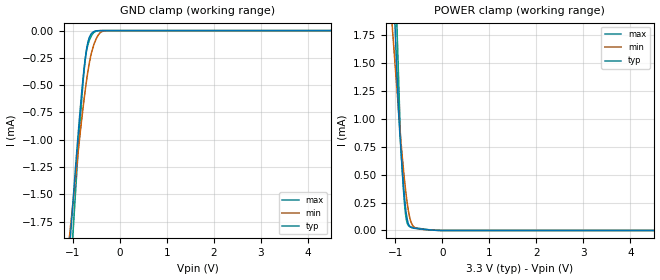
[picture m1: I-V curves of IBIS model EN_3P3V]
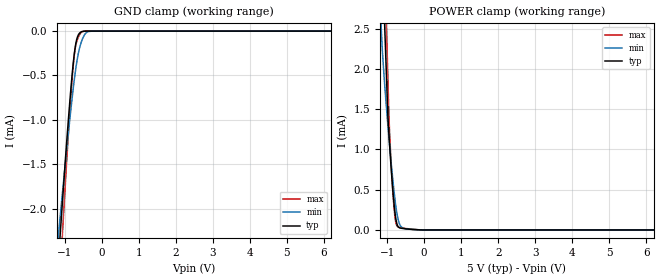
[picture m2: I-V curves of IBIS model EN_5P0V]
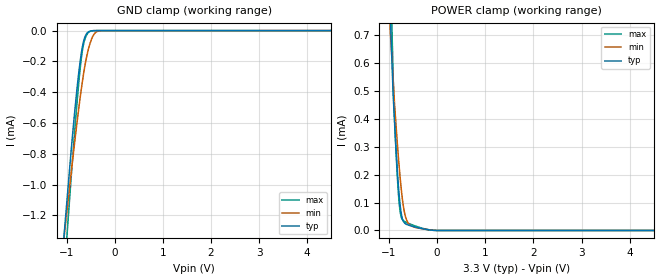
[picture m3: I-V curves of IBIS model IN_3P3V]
| Texas Instruments Incorporated
| Low-Power Quad-channel Digital Isolator
| Marketing part#   Voltage Range   Package-type   #pins/pkg drawing
| ISO7342CDW   3.0V - 5.5V   SOIC   16-pin DW
| ISO7342CDWR   3.0V - 5.5V   SOIC   16-pin DW
[IBIS Ver]   4.1
[File name]   iso7342.ibs
[File Rev]   1.1
[Date]   09/25/2014
[Source]   Model built from spectre simulations at:
   Texas Instruments Incorporated.
   Analog-eLab, HPA
   12500 TI Blvd
   Dallas, TX -75243
   For Support e-mail: elab_ibis@list.ti.com
[Notes]   Revision History
   Rev 1.1: 09/25/2014
   - Update OUT models to 3-state
   Rev 1.0: 07/25/2014
   - GND Clamp non monotonic for EN and IN input buffers
   - ccomp values are based on PVT settings:
   MIN: Low Voltage, High Temperature, Weak Process
   TYP: Nominal Voltage, Nominal Temperature, Nominal Process
   MAX: High Voltage, Low Temperature, Fast Process
   - C_comp although listed in numerical order of value are obtained from varying PVT conditions.
   For PVT conditions for each specific value, refer to the buffer description under respective [Model].
   IBIS model user is responsible for using appropriate C_comp to simulate for Signal Integrity.
[Disclaimer]  This model is designed as an aid for customers of Texas Instruments
 TI and its licensors and suppliers make no warranties, either expressed
 or implied, with respect to this  model, including the warranties of
 merchantability or fitness for a particular purpose.
 The model is provided solely on an "as is" basis. The entire risk as to
 its quality and performance is with the customer.
[Copyright] (C)Copyright 2014 Texas Instruments Incorporated.
   All rights reserved.
[Component]   ISO7342CDW
[Manufacturer]  Texas Instruments Incorporated
[Package]   |16-pin SOIC DW package
|   typ   min   max
R_pkg   0.1228   0.0822   0.1793
L_pkg   2.2157n   1.9245n   2.8571n
C_pkg   0.4645p   0.2145p   0.7510p
[Pin]   signal_name   model_name   R_pin   L_pin   C_pin
1   VCC1   POWER   0.09703  2.25823n  0.63889p
2   GND1   GND   0.10567  2.15194n  0.30706p
3   INA   IN   0.12889  1.99554n  0.21450p
4   INB   IN   0.12623  1.94755n  0.61276p
5   OUTC   OUT   0.12494  1.92646n  0.36666p
6   OUTD   OUT   0.14038  2.18765n  0.43235p
7   EN1   EN   0.17807  2.83638n  0.45904p
8   GND1   GND   0.08216  2.43955n  0.44498p
9   GND2   GND   0.10126  2.44074n  0.40934p
10   EN2   EN   0.17928  2.85707n  0.52717p
11   IND   IN   0.12883  1.99615n  0.50841p
12   INC   IN   0.12617  1.94399n  0.32633p
13   OUTB   OUT   0.12498  1.92454n  0.37783p
14   OUTA   OUT   0.14050  2.18615n  0.38097p
15   GND2   GND   0.08275  2.09014n  0.75096p
16   VCC2   POWER   0.09747  2.26909n  0.67439p
[Model Selector] IN
IN_3P3V   3.3V Input
IN_5P0V   5.0V Input
[Model Selector] EN
EN_3P3V   3.3V Input
EN_5P0V   5.0V Input
[Model Selector] OUT
OUT_3P3V   3.3V Output
OUT_5P0V   5.0V Output
| Models and submodels in the file (6): EN_3P3V (Input), EN_5P0V (Input), IN_3P3V (Input), IN_5P0V (Input), OUT_3P3V (3-state), OUT_5P0V (3-state)
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|   Model EN_3P3V
[Model]   EN_3P3V
Model_type   Input
Vinl = .8
Vinh = 2
|   typ   min   max
|   (nom PVT)   (slow PVT)   (fast PVT)
C_comp   0.161p   0.098p   0.252p
| Where   nom PVT is  Nominal Process, 3.3V, 27C
|   Fast PVT is Strong Process, 3.6V, -40C
|   Slow PVT is Weak Process, 3.0V, 150C
[Voltage Range]   3.3   3   3.6
[Temperature Range]   27   150   -40
[Power Clamp Reference]   3.3   3   3.6
[GND Clamp Reference]   0   0   0
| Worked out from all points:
|   GND clamp passes 1 mA (typ) near -0.90 V on its own axis
|   POWER clamp passes 1 mA (typ) near -0.92 V on its own axis
[GND Clamp]
|   Voltage   I(typ)   I(min)   I(max)
-3.3V     -16.02mA   -12.12mA   -20.07mA
-1.082V   -2.058mA   -1.927mA   -2.435mA
-933.9mV  -1.195mA   -1.301mA   -1.409mA
-815.1mV  -576.9uA   -823.1uA   -642.6uA
-775.5mV  -399.7uA   -677.1uA   -429.5uA
-735.9mV  -249.5uA   -540.6uA   -261.7uA
-696.3mV  -138.4uA   -417.2uA   -157.1uA
-656.7mV  -70.87uA   -311.6uA   -97.71uA
-547.8mV  -8.269uA   -122.2uA   -15.56uA
-438.9mV  -609.9nA   -28.59uA   -715.7nA
-300.3mV  -135.4nA   -1.693uA   -73.15nA
6.6V      0A         0A         0A
[POWER Clamp]
|   Voltage   I(typ)   I(min)   I(max)
-3.3V     37.87mA    27.97mA    46.61mA
-1.082V   2.59mA     1.912mA    3.362mA
-933.9mV  1.066mA    1.077mA    1.378mA
-894.3mV  792.6uA    854.2uA    848.9uA
-844.8mV  490.1uA    618.8uA    468.6uA
-795.3mV  245.9uA    408.6uA    190uA
-765.6mV  141.6uA    299.7uA    94.29uA
-735.9mV  76.12uA    208uA      52.02uA
-656.7mV  25.39uA    64.33uA    30.38uA
-518.1mV  15.3uA     15.27uA    20.19uA
-3.3mV    22.97nA    56.83nA    14.08nA
6.6V      0A         0A         0A
|   Model EN_5P0V
[Model]   EN_5P0V
Model_type   Input
Vinl = .8
Vinh = 2
|   typ   min   max
|   (nom PVT)   (slow PVT)   (fast PVT)
C_comp   0.173p   0.101p   0.247p
| Where   nom PVT is  Nominal Process, 5.0V, 27C
|   Fast PVT is Strong Process, 5.5V, -40C
|   Slow PVT is Weak Process, 4.5V, 150C
[Voltage Range]   5   4.5   5.5
[Temperature Range]   27   150   -40
[Power Clamp Reference]   5   4.5   5.5
[GND Clamp Reference]   0   0   0
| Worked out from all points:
|   GND clamp passes 1 mA (typ) near -0.90 V on its own axis
|   POWER clamp passes 1 mA (typ) near -0.92 V on its own axis
[GND Clamp]
|   Voltage   I(typ)   I(min)   I(max)
-5V       -26.85mA   -20.05mA   -33.83mA
-1.235V   -2.983mA   -2.6mA     -3.546mA
-1.13V    -2.354mA   -2.134mA   -2.795mA
-1.115V   -2.264mA   -2.068mA   -2.688mA
-1.055V   -1.904mA   -1.808mA   -2.259mA
-860mV    -799.2uA   -997uA     -914.7uA
-755mV    -317.8uA   -605uA     -335.4uA
-665mV    -81.82uA   -332uA     -109.5uA
-530mV    -5.449uA   -101.8uA   -10.68uA
-425mV    -437.8nA   -22.05uA   -447nA
-275mV    -117.8nA   -1.166uA   -60.6nA
10V       0A         0A         0A
[POWER Clamp]
|   Voltage   I(typ)   I(min)   I(max)
-5V       66.01mA    49.38mA    80.54mA
-1.235V   4.734mA    3.205mA    6.08mA
-1.13V    3.373mA    2.244mA    4.359mA
-1.085V   2.789mA    1.93mA     3.621mA
-1.055V   2.4mA      1.739mA    3.129mA
-1.025V   2.011mA    1.559mA    2.638mA
-980mV    1.427mA    1.304mA    1.9mA
-935mV    1.075mA    1.063mA    1.241mA
-845mV    491.9uA    621.1uA    470.4uA
-770mV    155.2uA    316.2uA    105.1uA
-650mV    24.69uA    59.36uA    30.24uA
10V       0A         0A         0A
|   Model IN_3P3V
[Model]   IN_3P3V
Model_type   Input
Vinl = .8
Vinh = 2
|   typ   min   max
|   (nom PVT)   (slow PVT)   (fast PVT)
C_comp   0.351p   0.323p   0.382p
| Where   nom PVT is  Nominal Process, 3.3V, 27C
|   Fast PVT is Strong Process, 3.6V, -40C
|   Slow PVT is Weak Process, 3.0V, 150C
[Voltage Range]   3.3   3   3.6
[Temperature Range]   27   150   -40
[Power Clamp Reference]   3.3   3   3.6
[GND Clamp Reference]   0   0   0
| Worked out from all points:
|   GND clamp passes 1 mA (typ) near -0.96 V on its own axis
|   POWER clamp passes 1 mA (typ) near -1.02 V on its own axis
[GND Clamp]
|   Voltage   I(typ)   I(min)   I(max)
-3.3V     -10.5mA    -8.177mA   -12.99mA
-1.082V   -1.445mA   -1.431mA   -1.727mA
-914.1mV  -816.9uA   -954.1uA   -998.5uA
-805.2mV  -448.8uA   -657.2uA   -556.2uA
-716.1mV  -199.7uA   -434.2uA   -244.8uA
-676.5mV  -117.1uA   -344.3uA   -142.2uA
-636.9mV  -59.87uA   -263.2uA   -75.98uA
-587.4mV  -22.32uA   -177.9uA   -31.66uA
-528mV    -5.765uA   -100.5uA   -8.109uA
-419.1mV  -436.4nA   -19.72uA   -339.2nA
-260.7mV  -145.3nA   -1.051uA   -79.88nA
6.6V      0A         0A         0A
[POWER Clamp]
|   Voltage   I(typ)   I(min)   I(max)
-3.3V     19.35mA    14.36mA    23.78mA
-1.082V   1.282mA    1.032mA    1.702mA
-914.1mV  486.5uA    539.1uA    550.7uA
-894.3mV  418uA      481uA      439.2uA
-844.8mV  262.9uA    353.4uA    248.9uA
-805.2mV  160.1uA    262.6uA    132.8uA
-775.5mV  100.8uA    201.4uA    76.11uA
-706.2mV  34.28uA    91.86uA    35.49uA
-627mV    21.23uA    34.25uA    27.78uA
-488.4mV  13.81uA    12.6uA     18.19uA
-3.3mV    4.025nA    17.39nA    2.182nA
6.6V      0A         0A         0A
